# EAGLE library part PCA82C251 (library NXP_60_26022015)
CAN transceiver for 24 V systems The PCA82C251 is the interface between a CAN protocol controller and the physical bus. The device provides differential transmit capability to the bus and differential receive capability to the CAN controller AAL Eindhoven MK
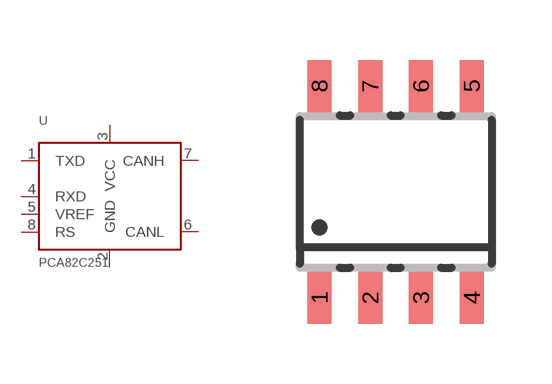
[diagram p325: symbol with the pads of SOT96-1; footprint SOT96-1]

Designator prefix U

## PCA82C251T  [SOT96-1]
1  TXD  out
2  GND
3  VCC
4  RXD
5  VREF  pwr
6  CANL
7  CANH
8  RS  pas

## Footprint SOT96-1 (pad centres in mm)
SOT96-1 SO8: plastic small outline package; 8 leads; body width 3.9 mm JEDEC: MS-012 IEC: 076E03
smd 0.6 x 1.3: 1 -1.905,-2.65; 2 -0.635,-2.65; 3 0.635,-2.65; 4 1.905,-2.65; 5 1.905,2.65; 6 0.635,2.65; 7 -0.635,2.65; 8 -1.905,2.65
